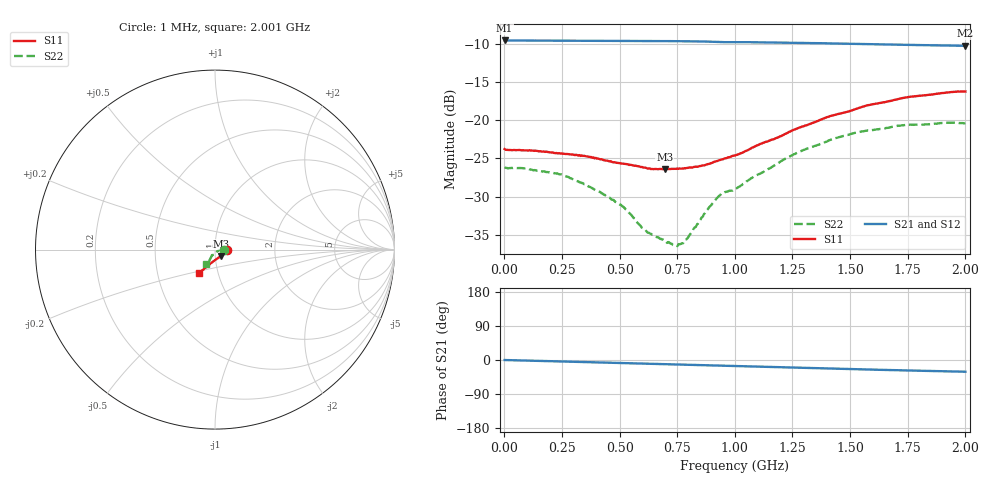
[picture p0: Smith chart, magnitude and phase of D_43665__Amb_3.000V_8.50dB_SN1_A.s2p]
! device id: 43665_
! dir: \\malibu\benchdata\1_engineers\tn_data\43665_75ohm\new\sparar\43665_\amb\3p000v\8p50db
! Serial: 1
! Insertion: A
! Temp: Amb
! VDD: 3.000V
! Attenuation Step: 8.50dB
! IDD: 1.453167e+00mA
! FILE NAME
! DATE 03-27-2009 08:35:26
! CORRECTED  DATA
#  Hz  S  RI  R  75
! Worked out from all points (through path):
!   401 points, 1 MHz to 2.001 GHz, reference 75 ohm
!   highest |S21| = -9.54 dB at 1 MHz (marker M1); lowest = -10.2 dB at 2.001 GHz (marker M2)
!   group delay of S21, straight-line fit = 43.8 ps
!   lowest |S11| = -26.4 dB at 696 MHz (marker M3), VSWR 1.10, Z = 79.7 - j5.72 ohm
!   |S11| at or under -10 dB: start of sweep to end of sweep
!   |S22| runs from -36.5 to -20.3 dB; largest |S21 - S12| = 0.0013
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1000000  0.0647 -0.000981  0.3335 -0.000456  0.3338 -0.000429  0.0492 -0.000527
8.6e7  0.0634 -0.00375  0.3329 -0.00769  0.3331 -0.00773  0.0484 0.00154
2.21e8  0.0602 -0.00888  0.3322 -0.0199  0.3324 -0.02  0.0448 0.0022
3.36e8  0.0569 -0.0144  0.3311 -0.0304  0.3312 -0.0304  0.0387 0.00291
5.06e8  0.0465 -0.0235  0.3286 -0.0461  0.3286 -0.0461  0.0278 -0.0013
6.06e8  0.0392 -0.0293  0.3262 -0.0549  0.3262 -0.0551  0.0188 -0.00484
6.71e8  0.0336 -0.0341  0.3248 -0.061  0.3248 -0.061  0.0146 -0.00859
6.96e8  0.0316 -0.0358  0.3242 -0.0633  0.3241 -0.0633  0.0132 -0.00968
7.41e8  0.0279 -0.0391  0.3229 -0.0676  0.323 -0.0676  0.00916 -0.012
7.71e8  0.0251 -0.0411  0.3219 -0.0705  0.322 -0.0704  0.00622 -0.0143
8.01e8  0.0224 -0.0435  0.3209 -0.0733  0.3209 -0.0733  0.00361 -0.017
8.76e8  0.0141 -0.0492  0.3178 -0.0805  0.3179 -0.0804  -0.0023 -0.0253
9.31e8  0.00767 -0.0541  0.3145 -0.085  0.3147 -0.0847  -0.00945 -0.0304
9.51e8  0.00562 -0.0553  0.3135 -0.0861  0.3137 -0.0859  -0.0129 -0.0308
1.001e9  0.000592 -0.0587  0.3124 -0.0892  0.3126 -0.089  -0.0172 -0.0307
1.216e9  -0.0244 -0.0772  0.3042 -0.1077  0.3046 -0.1077  -0.0256 -0.0493
1.336e9  -0.0373 -0.0881  0.2983 -0.1169  0.2988 -0.1168  -0.0312 -0.0592
1.411e9  -0.0459 -0.0956  0.2944 -0.123  0.295 -0.1232  -0.0325 -0.0664
1.521e9  -0.057 -0.1032  0.2885 -0.1302  0.289 -0.1306  -0.0389 -0.0729
1.671e9  -0.0698 -0.1138  0.2807 -0.1399  0.2807 -0.1406  -0.0424 -0.079
1.761e9  -0.0759 -0.1205  0.2759 -0.1453  0.276 -0.1463  -0.0437 -0.0828
2.001e9  -0.0867 -0.1276  0.2637 -0.1582  0.2626 -0.159  -0.0484 -0.0821
